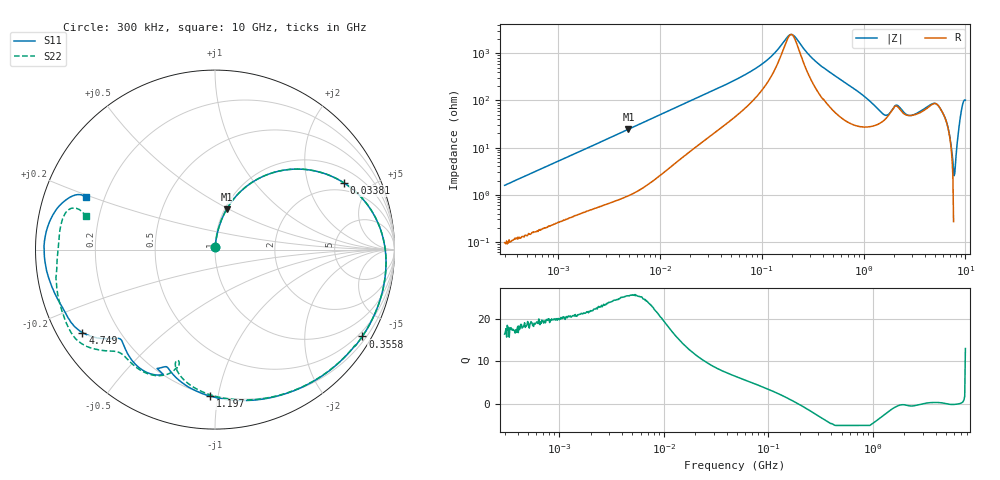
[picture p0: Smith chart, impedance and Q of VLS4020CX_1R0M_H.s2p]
! S-Parameter Data Generated by TDK Corporation
! Copyright(C) 2024 TDK Corporation.
! All Rights Reserved.
! TDK P/N: VLS4020CX-1R0M-H (SMD / SMT Inductor (Coil))
! Property: L=1uH at 1MHz
! Size(LxWxT): 4x4x2mm
! Model Type: s2p (Touchstone File Format Version 1.0)
! Frequency: DC=Yes Start=0.3MHz Stop=10000MHz 802points Log-sweep
! Model Generated on May 28, 2024
! Terms and conditions regarding TDK Simulation Models:
! 1)This simulation model is being provided solely for informational
!  purposes. Please refer to the specifications of the products in
!  terms of detailed characteristics of such products.
! 2)In no event shall TDK Corporation of any of its subsidiaries be
!  liable for any loss or damage arising, directly or indirectly,
!  from any information contained in this simulation model, including,
!  but not limited to loss or damages arising from any inaccuracies,
!  omissions or errors in connection with such information.
! 3)Any and all copyrights on this simulation model are owned by
!  TDK Corporation.  Duplication or redistribution of this simulation
!  model without prior written permission from TDK Corporation
!  is prohibited.
! 4)This simulation model is subject to any modification or change
!  without any prior notice.
! 5)Neither TDK Corporation nor any of its subsidiaries shall make any
!  warranty, express or implied, including but not limited to the
!  correctness, implied warranties of merchantability and fitness for
!  a particular purpose with respect to this simulation models.
! 6)The use of this simulation model shall be deemed to have consented
!  to the terms and conditions hereof.
! Port Assignments:
!  1 ---@@@--- 2
! Applicable Conditions:
!  Temperature = 25 degC
!  DC Bias Current = 0 A
!  Small Signal Operation
# Hz S MA R 50
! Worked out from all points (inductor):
!   801 points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, 300 kHz to 10 GHz, reference 50 ohm
!   read as one part in series: L = 836 nH near 318.3 kHz
!   highest Q = 25.5 at 4.921 MHz (marker M1), where L = 788 nH
!   self-resonance near 194.7 MHz
!   S11 on the Smith chart (normalised r, x): 300 kHz: 1.00, +0.03; 33.81 MHz: 1.59, +3.41; 355.8 MHz: 0.35, -3.64; 1.197 GHz: 0.19, -0.95; 4.749 GHz: 0.07, -0.29; 10 GHz: 0.13, +0.19
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300000  0.01562 85.5  0.999 -0.9  0.9988 -0.9  0.01571 85.6
1713600  0.08525 82.3  0.9923 -5.0  0.9923 -5.0  0.08521 82.3
4920797  0.2325 74.0  0.9635 -13.7  0.9634 -13.7  0.2325 74.0
9671944  0.4193 61.7  0.8868 -25.4  0.8868 -25.4  0.4192 61.7
1.831589e7  0.6386 44.6  0.7192 -40.7  0.7192 -40.7  0.6385 44.7
3.38066e7  0.8084 27.4  0.4972 -55.5  0.4972 -55.5  0.8084 27.5
5.477226e7  0.8899 15.6  0.331 -64.8  0.331 -64.8  0.89 15.6
1.112655e8  0.9476 0.4  0.1364 -70.8  0.1365 -70.8  0.9476 0.5
1.923314e8  0.9613 -12.0  0.03804 -15.8  0.03806 -15.8  0.9612 -11.8
3.126428e8  0.9571 -26.0  0.1147 46.3  0.1147 46.3  0.9572 -25.6
3.558009e8  0.9529 -30.5  0.1447 45.8  0.1447 45.8  0.9532 -30.0
6.904357e8  0.9037 -59.4  0.3082 23.2  0.3082 23.2  0.9037 -58.7
1.196827e9  0.8167 -91.9  0.4216 -13.1  0.4217 -13.1  0.8126 -91.1
1.50342e9  0.7538 -105.6  0.4426 -35.1  0.4428 -35.1  0.7346 -104.8
1.767019e9  0.7074 -112.1  0.4127 -56.5  0.4131 -56.5  0.6569 -109.2
2.264206e9  0.7833 -120.8  0.2841 -67.4  0.2841 -67.6  0.7753 -115.1
3.261479e9  0.7286 -137.2  0.2522 -105.3  0.2519 -105.4  0.7854 -133.4
4.749267e9  0.8713 -147.9  0.09499 -135.4  0.09471 -135.4  0.903 -143.9
6.333834e9  0.9146 -161.3  0.0747 -129.6  0.07466 -129.5  0.9193 -157.8
7.652089e9  0.9519 -179.4  0.05754 -146.5  0.05759 -146.3  0.8818 -176.1
9.105558e9  0.8807 162.1  0.03488 -149.3  0.03502 -149.2  0.8585 166.3
1e10  0.7778 158.0  0.03315 -134.6  0.03324 -134.6  0.7436 165.5
